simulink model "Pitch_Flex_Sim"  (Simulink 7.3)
settings: Solver=ode45  StartTime=0.0  StopTime=140  RelTol=1e-3
InitFcn:
  | r2d= 180/pi; d2r=1/r2d; Ts=0.04;
  | [Apf,Bpf,Cpf,Dpf]= pitch_vehi_flex;              % Shuttle Ascent, Max_Q, T=55 sec, Flex Pitch Vehicle with Slosh and TWD
  | [Aac,Bac,Cac,Dac]= ssme_actuator;                % Shuttle Main Engine Actuator
  | [Asb,Bsb,Csb,Dsb]= srb_actuator;                 % Solid Rocket Booster Actuator
  | [Afc,Bfc,Cfc,Dfc]= pitch_fcs;                    % Pitch Axis Discrete FCS
  | [Apl,Bpl,Cpl,Dpl]= pitch_plant_s;                % Pitch Plant (Flex Vehicle, Actuators, TVC, TWD)
  | [Apz,Bpz,Cpz,Dpz]= pitch_plant_z;                % Pitch Plant Discrete
  | [Aol,Bol,Col,Dol]= open_loop;                    % Open-Loop Pitch (Plant Model + Controller)
  | [Acl,Bcl,Ccl,Dcl]= closed_loop;                  % Closed Loop (Plant Model + Controller)
StopFcn:
  | Pl
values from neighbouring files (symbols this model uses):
  Aac = [    [actuator_srb.m]    (also in actuator_ssme.m; actuators_5s.m; actuators_5z.m)
  Bac = [    [actuator_srb.m]    (also in actuator_ssme.m; actuators_5s.m; actuators_5z.m)
  Cac = [    [actuator_srb.m]    (also in actuator_ssme.m; actuators_5s.m; actuators_5z.m)
  Dac = [    [actuator_srb.m]    (also in actuator_ssme.m; actuators_5s.m; actuators_5z.m)
undefined symbols (not defined in the file or in its folder): Afc, Apf, Asb, Bfc, Bpf, Bsb, Cfc, Cpf, Csb, Dfc, Dpf, Dsb

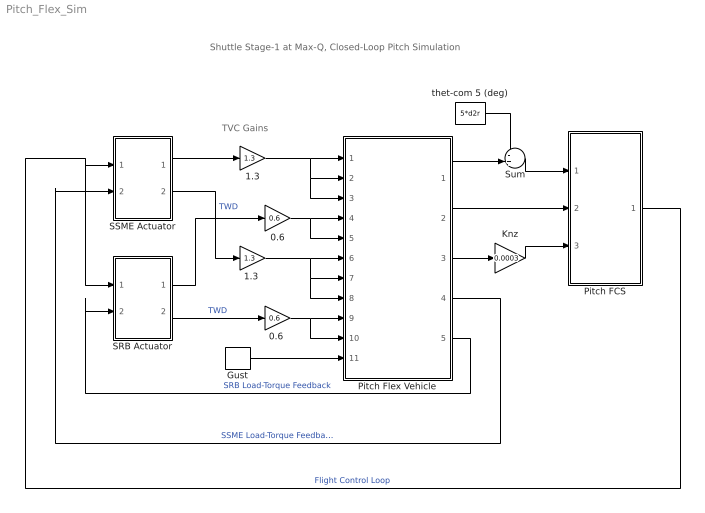
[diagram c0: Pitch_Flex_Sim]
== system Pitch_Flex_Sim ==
  note: TVC Gains
  note: Shuttle Stage-1 at Max-Q, Closed-Loop Pitch Simulation
  0.6 : Gain  Gain=0.6  ParameterDataType=sfix(16)  ParameterScaling=2^0  OutDataType=sfix(16)  OutScaling=2^0
  "0.6 " : Gain  Gain=0.6  ParameterDataType=sfix(16)  ParameterScaling=2^0  OutDataType=sfix(16)  OutScaling=2^0
  1.3 : Gain  Gain=1.3  ParameterDataType=sfix(16)  ParameterScaling=2^0  OutDataType=sfix(16)  OutScaling=2^0
  "1.3 " : Gain  Gain=1.3  ParameterDataType=sfix(16)  ParameterScaling=2^0  OutDataType=sfix(16)  OutScaling=2^0
  Gust : DiscretePulseGenerator  PulseType=Time based  Amplitude=30  Period=200  PulseWidth=2  PhaseDelay=0.2  SampleTime=1
  Knz : Gain  Gain=0.0003  ParameterDataType=sfix(16)  ParameterScaling=2^0  OutDataType=sfix(16)  OutScaling=2^0
  Pitch FCS : Subsystem
  Pitch Flex Vehicle : Subsystem
  SRB Actuator : Subsystem
  SSME Actuator : Subsystem
  Sum : Sum  Inputs=-+|  OutDataType=sfix(16)  OutScaling=2^0
  thet-com 5 (deg) : Constant  Value=5*d2r  OutDataType=sfix(16)  OutScaling=2^0
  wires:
  SSME Actuator/1(dy) -> 1.3/1
  Pitch FCS/1(DQ_TVC) -> SSME Actuator/1(dy-com), SRB Actuator/1(dy-com)  "Flight Control Loop"
  "1.3 "/1 -> Pitch Flex Vehicle/6(dydd1), Pitch Flex Vehicle/7(dydd2), Pitch Flex Vehicle/8(dydd3)
  "0.6 "/1 -> Pitch Flex Vehicle/9(dydd4), Pitch Flex Vehicle/10(dydd5)
  Pitch Flex Vehicle/2(q-flx) -> Pitch FCS/2(q)
  Pitch Flex Vehicle/3(Nz) -> Knz/1
  Knz/1 -> Pitch FCS/3(Nz)
  Pitch Flex Vehicle/1(theta) -> Sum/2
  Sum/1 -> Pitch FCS/1(theta)
  thet-com 5 (deg)/1 -> Sum/1
  SRB Actuator/1(dy) -> 0.6/1
  SRB Actuator/2(dy-dd) -> "0.6 "/1  "TWD"
  SSME Actuator/2(dy-dd) -> "1.3 "/1  "TWD"
  Pitch Flex Vehicle/5(TLy_srb) -> SRB Actuator/2(TL)  "SRB Load-Torque Feedback"
  Pitch Flex Vehicle/4(TLy_sme) -> SSME Actuator/2(TL)  "SSME Load-Torque Feedback"
  1.3/1 -> Pitch Flex Vehicle/1(dy1), Pitch Flex Vehicle/2(dy2), Pitch Flex Vehicle/3(dy3)
  0.6/1 -> Pitch Flex Vehicle/4(dy4), Pitch Flex Vehicle/5(dy5)
  Gust/1 -> Pitch Flex Vehicle/11(WG)

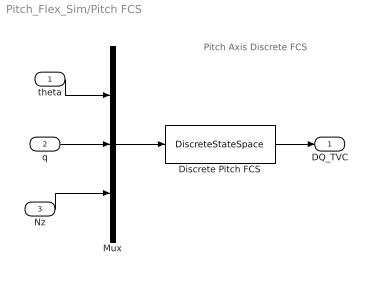
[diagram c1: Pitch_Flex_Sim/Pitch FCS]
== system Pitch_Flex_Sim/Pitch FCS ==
  note: Pitch Axis Discrete FCS
  theta : Inport  OutDataType=sfix(16)  OutScaling=2^0
  q : Inport  Port=2  OutDataType=sfix(16)  OutScaling=2^0
  Nz : Inport  Port=3  OutDataType=sfix(16)  OutScaling=2^0
  Discrete Pitch FCS : DiscreteStateSpace  A=Afc  B=Bfc  C=Cfc  D=Dfc  SampleTime=0.04
  Mux : Mux  Inputs=3
  DQ_TVC : Outport  OutDataType=sfix(16)  OutScaling=2^0
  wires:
  Discrete Pitch FCS/1 -> DQ_TVC/1
  theta/1 -> Mux/1
  q/1 -> Mux/2
  Nz/1 -> Mux/3
  Mux/1 -> Discrete Pitch FCS/1

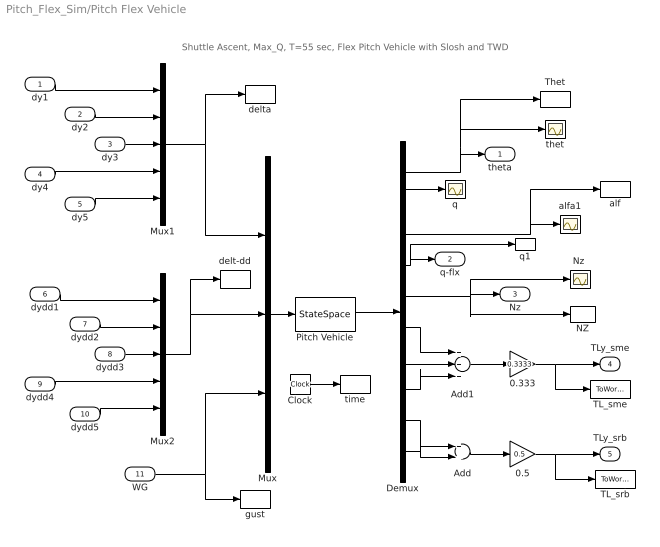
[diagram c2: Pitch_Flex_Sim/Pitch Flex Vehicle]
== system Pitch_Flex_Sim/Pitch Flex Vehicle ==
  note: Shuttle Ascent, Max_Q, T=55 sec, Flex Pitch Vehicle with Slosh and TWD
  dy1 : Inport  OutDataType=sfix(16)  OutScaling=2^0
  dy2 : Inport  Port=2  OutDataType=sfix(16)  OutScaling=2^0
  dy3 : Inport  Port=3  OutDataType=sfix(16)  OutScaling=2^0
  dy4 : Inport  Port=4  OutDataType=sfix(16)  OutScaling=2^0
  dy5 : Inport  Port=5  OutDataType=sfix(16)  OutScaling=2^0
  dydd1 : Inport  Port=6  OutDataType=sfix(16)  OutScaling=2^0
  dydd2 : Inport  Port=7  OutDataType=sfix(16)  OutScaling=2^0
  dydd3 : Inport  Port=8  OutDataType=sfix(16)  OutScaling=2^0
  dydd4 : Inport  Port=9  OutDataType=sfix(16)  OutScaling=2^0
  dydd5 : Inport  Port=10  OutDataType=sfix(16)  OutScaling=2^0
  WG : Inport  Port=11  OutDataType=sfix(16)  OutScaling=2^0
  0.333 : Gain  Gain=0.3333  ParameterDataType=sfix(16)  ParameterScaling=2^0  OutDataType=sfix(16)  OutScaling=2^0
  0.5 : Gain  Gain=0.5  ParameterDataType=sfix(16)  ParameterScaling=2^0  OutDataType=sfix(16)  OutScaling=2^0
  Add : Sum  OutDataType=sfix(16)  OutScaling=2^-10
  Add1 : Sum  Inputs=+++  OutDataType=sfix(16)  OutScaling=2^-10
  Clock : Clock
  Demux : Demux  Outputs=10
  Mux : Mux  Inputs=[5 5 1]
  Mux1 : Mux  Inputs=5
  Mux2 : Mux  Inputs=5
  NZ : ToWorkspace  VariableName=Nz  SampleTime=-1  SaveFormat=Array
  "Nz " : Scope
  Pitch Vehicle : StateSpace  A=Apf  B=Bpf  C=Cpf  D=Dpf
  TL_sme : ToWorkspace  VariableName=TL_sme  SampleTime=-1  SaveFormat=Array
  TL_srb : ToWorkspace  VariableName=TL_srb  SampleTime=-1  SaveFormat=Array
  Thet : ToWorkspace  VariableName=theta  SampleTime=-1  SaveFormat=Array
  alf : ToWorkspace  VariableName=alpha  SampleTime=-1  SaveFormat=Array
  alfa1 : Scope
  delt-dd : ToWorkspace  VariableName=deltdd  SampleTime=-1  SaveFormat=Array
  delta : ToWorkspace  VariableName=delta  SampleTime=-1  SaveFormat=Array
  gust : ToWorkspace  VariableName=Gust  SampleTime=-1  SaveFormat=Array
  q : Scope
  q1 : ToWorkspace  VariableName=q  SampleTime=-1  SaveFormat=Array
  thet : Scope
  time : ToWorkspace  VariableName=time  SampleTime=-1  SaveFormat=Array
  theta : Outport  OutDataType=sfix(16)  OutScaling=2^0
  q-flx : Outport  Port=2  OutDataType=sfix(16)  OutScaling=2^0
  Nz : Outport  Port=3  OutDataType=sfix(16)  OutScaling=2^0
  TLy_sme : Outport  Port=4  OutDataType=sfix(16)  OutScaling=2^0
  TLy_srb : Outport  Port=5  OutDataType=sfix(16)  OutScaling=2^0
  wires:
  Pitch Vehicle/1 -> Demux/1
  Mux/1 -> Pitch Vehicle/1
  Demux/2 -> q/1
  Demux/3 -> alfa1/1, alf/1
  WG/1 -> gust/1, Mux/3
  Demux/1 -> theta/1, thet/1, Thet/1
  Demux/5 -> Nz/1, "Nz "/1, NZ/1
  Demux/4 -> q-flx/1, q1/1
  Clock/1 -> time/1
  dy1/1 -> Mux1/1
  dy2/1 -> Mux1/2
  dy4/1 -> Mux1/4
  dy5/1 -> Mux1/5
  dy3/1 -> Mux1/3
  dydd1/1 -> Mux2/1
  dydd2/1 -> Mux2/2
  dydd3/1 -> Mux2/3
  dydd4/1 -> Mux2/4
  dydd5/1 -> Mux2/5
  Mux2/1 -> Mux/2, delt-dd/1
  Mux1/1 -> Mux/1, delta/1
  Demux/7 -> Add1/2
  Demux/8 -> Add1/3
  Demux/6 -> Add1/1
  Demux/10 -> Add/2
  Demux/9 -> Add/1
  Add1/1 -> 0.333/1
  Add/1 -> 0.5/1
  0.333/1 -> TLy_sme/1, TL_sme/1
  0.5/1 -> TLy_srb/1, TL_srb/1

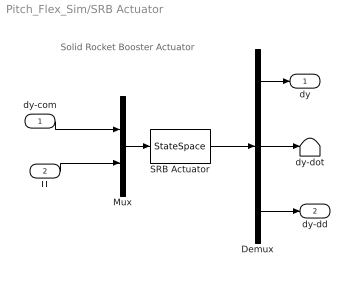
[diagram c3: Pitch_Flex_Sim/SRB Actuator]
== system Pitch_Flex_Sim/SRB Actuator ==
  note: Solid Rocket Booster Actuator
  dy-com : Inport  PortDimensions=1  OutDataType=sfix(16)  OutScaling=2^0
  TL : Inport  Port=2  OutDataType=sfix(16)  OutScaling=2^0
  Demux : Demux  Outputs=3
  Mux : Mux  Inputs=2
  SRB Actuator : StateSpace  A=Asb  B=Bsb  C=Csb  D=Dsb
  dy-dot : Terminator
  dy : Outport  OutDataType=sfix(16)  OutScaling=2^0
  dy-dd : Outport  Port=2  OutDataType=sfix(16)  OutScaling=2^0
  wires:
  Demux/3 -> dy-dd/1
  Demux/2 -> dy-dot/1
  TL/1 -> Mux/2
  dy-com/1 -> Mux/1
  Demux/1 -> dy/1
  Mux/1 -> SRB Actuator/1
  SRB Actuator/1 -> Demux/1

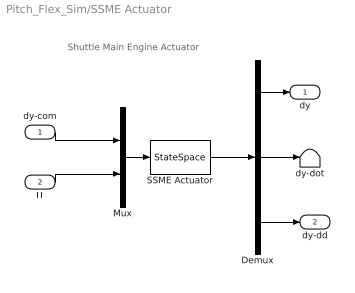
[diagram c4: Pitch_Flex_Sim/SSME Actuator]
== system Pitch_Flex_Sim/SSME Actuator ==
  note: Shuttle Main Engine Actuator
  dy-com : Inport  PortDimensions=1  OutDataType=sfix(16)  OutScaling=2^0
  TL : Inport  Port=2  OutDataType=sfix(16)  OutScaling=2^0
  Demux : Demux  Outputs=3
  Mux : Mux  Inputs=2
  SSME Actuator : StateSpace  A=Aac  B=Bac  C=Cac  D=Dac
  dy-dot : Terminator
  dy : Outport  OutDataType=sfix(16)  OutScaling=2^0
  dy-dd : Outport  Port=2  OutDataType=sfix(16)  OutScaling=2^0
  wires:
  Demux/3 -> dy-dd/1
  Demux/2 -> dy-dot/1
  TL/1 -> Mux/2
  dy-com/1 -> Mux/1
  Demux/1 -> dy/1
  Mux/1 -> SSME Actuator/1
  SSME Actuator/1 -> Demux/1
